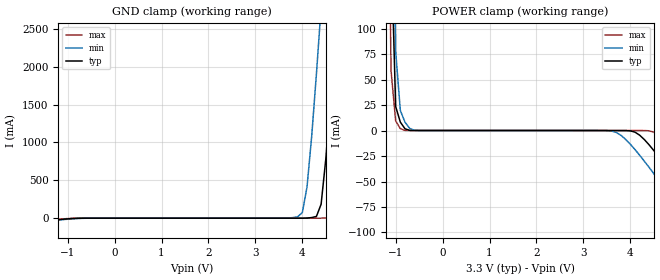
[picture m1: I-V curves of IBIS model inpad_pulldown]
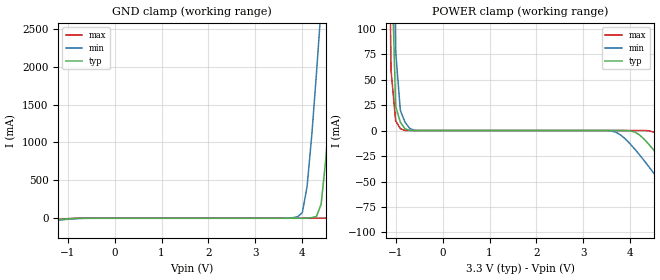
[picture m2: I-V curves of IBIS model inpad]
[IBIS Ver]   2.1
[File Name]   dac2904y.ibs
[File Rev]   1.1
[Source]   Preliminary IBIS Model Generated Manually
[Notes]
   Package information estimated
[Disclaimer]   This information is for modeling purposes only
[Copyright]   (c) 2004, Texas Instruments Inc.
[Component]   TQFP48
[Manufacturer]   Texas Instruments
[Package]
| Variable   Typ   Min   Max
R_pkg   0.1   0.1   0.1
L_pkg   3.0nH   3.0nH   3.0nH
C_pkg   3.0pF   3.0pF   3.0pF
[Pin]   signal_name   model_name   R_pin  L_pin   C_pin
   1   bit13_1   inpad   0.1   3.0nH   3.0pF
   2   bit12_1   inpad   0.1   3.0nH   3.0pF
   3   bit11_1   inpad   0.1   3.0nH   3.0pF
   4   bit10_1   inpad   0.1   3.0nH   3.0pF
   5   bit9_1   inpad   0.1   3.0nH   3.0pF
   6   bit8_1   inpad   0.1   3.0nH   3.0pF
   7   bit7_1   inpad   0.1   3.0nH   3.0pF
   8   bit6_1   inpad   0.1   3.0nH   3.0pF
   9   bit5_1   inpad   0.1   3.0nH   3.0pF
   10   bit4_1   inpad   0.1   3.0nH   3.0pF
   11   bit3_1   inpad   0.1   3.0nH   3.0pF
   12   bit2_1   inpad   0.1   3.0nH   3.0pF
   13   bit1_1   inpad   0.1   3.0nH   3.0pF
   14   bit0_1   inpad   0.1   3.0nH   3.0pF
   15   dgnd   GND   0.1   3.0nH   3.0pF
   16   vd   POWER   0.1   3.0nH   3.0pF
   17   wrt1   inpad   0.1   3.0nH   3.0pF
   18   clk1   inpad   0.1   3.0nH   3.0pF
   19   clk2   inpad   0.1   3.0nH   3.0pF
   20   wrt2   inpad   0.1   3.0nH   3.0pF
   21   dgnd   GND   0.1   3.0nH   3.0pF
   22   vd   POWER   0.1   3.0nH   3.0pF
   23   bit13_2   inpad   0.1   3.0nH   3.0pF
   24   bit12_2   inpad   0.1   3.0nH   3.0pF
   25   bit11_2   inpad   0.1   3.0nH   3.0pF
   26   bit10_2   inpad   0.1   3.0nH   3.0pF
   27   bit9_2   inpad   0.1   3.0nH   3.0pF
   28   bit8_2   inpad   0.1   3.0nH   3.0pF
   29   bit7_2   inpad   0.1   3.0nH   3.0pF
   30   bit6_2   inpad   0.1   3.0nH   3.0pF
   31   bit5_2   inpad   0.1   3.0nH   3.0pF
   32   bit4_2   inpad   0.1   3.0nH   3.0pF
   33   bit3_2   inpad   0.1   3.0nH   3.0pF
   34   bit2_2   inpad   0.1   3.0nH   3.0pF
   35   bit1_2   inpad   0.1   3.0nH   3.0pF
   36   bit0_2   inpad   0.1   3.0nH   3.0pF
   37   pd   inpad_pulldown   0.1   3.0nH   3.0pF
   38   agnd   GND   0.1   3.0nH   3.0pF
|  39   iout2   0.1   3.0nH   3.0pF
|  40   iout2b   0.1   3.0nH   3.0pF
|  41   fsa2   0.1   3.0nH   3.0pF
|  42   gset   0.1   3.0nH   3.0pF
|  43   refin   0.1   3.0nH   3.0pF
|  44   fsa1   0.1   3.0nH   3.0pF
|  45   iout1b   0.1   3.0nH   3.0pF
|  46   iout1   0.1   3.0nH   3.0pF
   47   va   POWER   0.1   3.0nH   3.0pF
|  48   nc   0.1   3.0nH   3.0pF
| End of package information
| Models and submodels in the file (2): inpad_pulldown (Input), inpad (Input)
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|   Model inpad_pulldown
[Model]   inpad_pulldown
Model_type   Input
Polarity   Non-Inverting
| signals   A, Y
Vinl = 0.8V
Vinh = 2.4V
|   typ   min   max
C_comp   1.5p   1.5p   1.5p
|   typ   min   max
[Temperature Range]   25   -40.0   100
|   typ   min   max
[Voltage Range]   3.30V   3.00V   3.60V
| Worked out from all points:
|   GND clamp passes 1 mA (typ) near -0.75 V on its own axis
|   POWER clamp passes 1 mA (typ) near -0.76 V on its own axis
[GND_clamp]
|   Voltage   I(typ)   I(min)   I(max)
-3.3V     -158.5mA   -161.4mA   -157.9mA
3.9V      30.58uA    19.49mA    62.29uA
4V        103.5uA    74.53mA    62.3uA
4.1V      1.681mA    413.8mA    62.32uA
4.3V      23.39mA    1.904A     62.62uA
4.4V      184.2mA    2.782A     94.62uA
4.6V      1.593A     4.618A     9.612mA
4.7V      2.479A     5.558A     57.33mA
4.8V      3.397A     6.507A     539.4mA
5V        5.282A     8.424A     2.248A
5.1V      6.239A     9.389A     3.179A
6.6V      20.93A     24.09A     17.83A
[POWER_clamp]
|   Voltage   I(typ)   I(min)   I(max)
-3.3V     20.93A     21.13A     20.8A
-1.2V     781.9mA    1.092A     542.9mA
-1.1V     188.9mA    420.5mA    59.9mA
-1V       23.64mA    77.91mA    9.61mA
-900mV    8.218mA    19.62mA    1.853mA
-800mV    1.699mA    8.086mA    96.45uA
3.6V      -8.708uA   -506.3uA   -1.736uA
4.5V      -19.54mA   -42.24mA   -1.61mA
5.4V      -76.76mA   -100.7mA   -53.85mA
5.8V      -103.7mA   -127.5mA   -81.04mA
6.1V      -124.1mA   -147.8mA   -101.8mA
6.6V      -158.5mA   -182mA     -136.7mA
|   Model inpad
[Model]   inpad
Model_type   Input
Polarity   Non-Inverting
| signals   A, Y
Vinl = 0.8V
Vinh = 2.4V
|   typ   min   max
C_comp   1.5p   1.5p   1.5p
|   typ   min   max
[Temperature Range]   25   -40.0   100
|   typ   min   max
[Voltage Range]   3.30V   3.00V   3.60V
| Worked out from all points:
|   GND clamp passes 1 mA (typ) near -0.76 V on its own axis
|   POWER clamp passes 1 mA (typ) near -0.76 V on its own axis
[GND_clamp]
|   Voltage   I(typ)   I(min)   I(max)
-3.3V     -157.3mA   -160.6mA   -155.8mA
3.9V      2.185uA    19.49mA    1.051nA
4V        79.64uA    74.52mA    1.095nA
4.1V      1.669mA    413.8mA    1.348nA
4.3V      23.39mA    1.904A     331nA
4.4V      184.2mA    2.782A     36.42uA
4.6V      1.593A     4.618A     9.596mA
4.7V      2.479A     5.558A     57.32mA
4.8V      3.397A     6.507A     539.4mA
5V        5.282A     8.424A     2.248A
5.1V      6.239A     9.389A     3.178A
6.6V      20.93A     24.09A     17.83A
[POWER_clamp]
|   Voltage   I(typ)   I(min)   I(max)
-3.3V     20.93A     21.13A     20.8A
-1.2V     781.9mA    1.092A     542.9mA
-1.1V     188.9mA    420.5mA    59.89mA
-1V       23.63mA    77.91mA    9.594mA
-900mV    8.211mA    19.62mA    1.826mA
-800mV    1.687mA    8.083mA    38.4uA
3.6V      -6.621nA   -469.2uA   -1.287nA
4.5V      -19.27mA   -41.88mA   -1.53mA
5.4V      -76.1mA    -100mA     -53mA
5.8V      -102.8mA   -126.8mA   -79.87mA
6.1V      -123.2mA   -147mA     -100.4mA
6.6V      -157.3mA   -181mA     -134.9mA
